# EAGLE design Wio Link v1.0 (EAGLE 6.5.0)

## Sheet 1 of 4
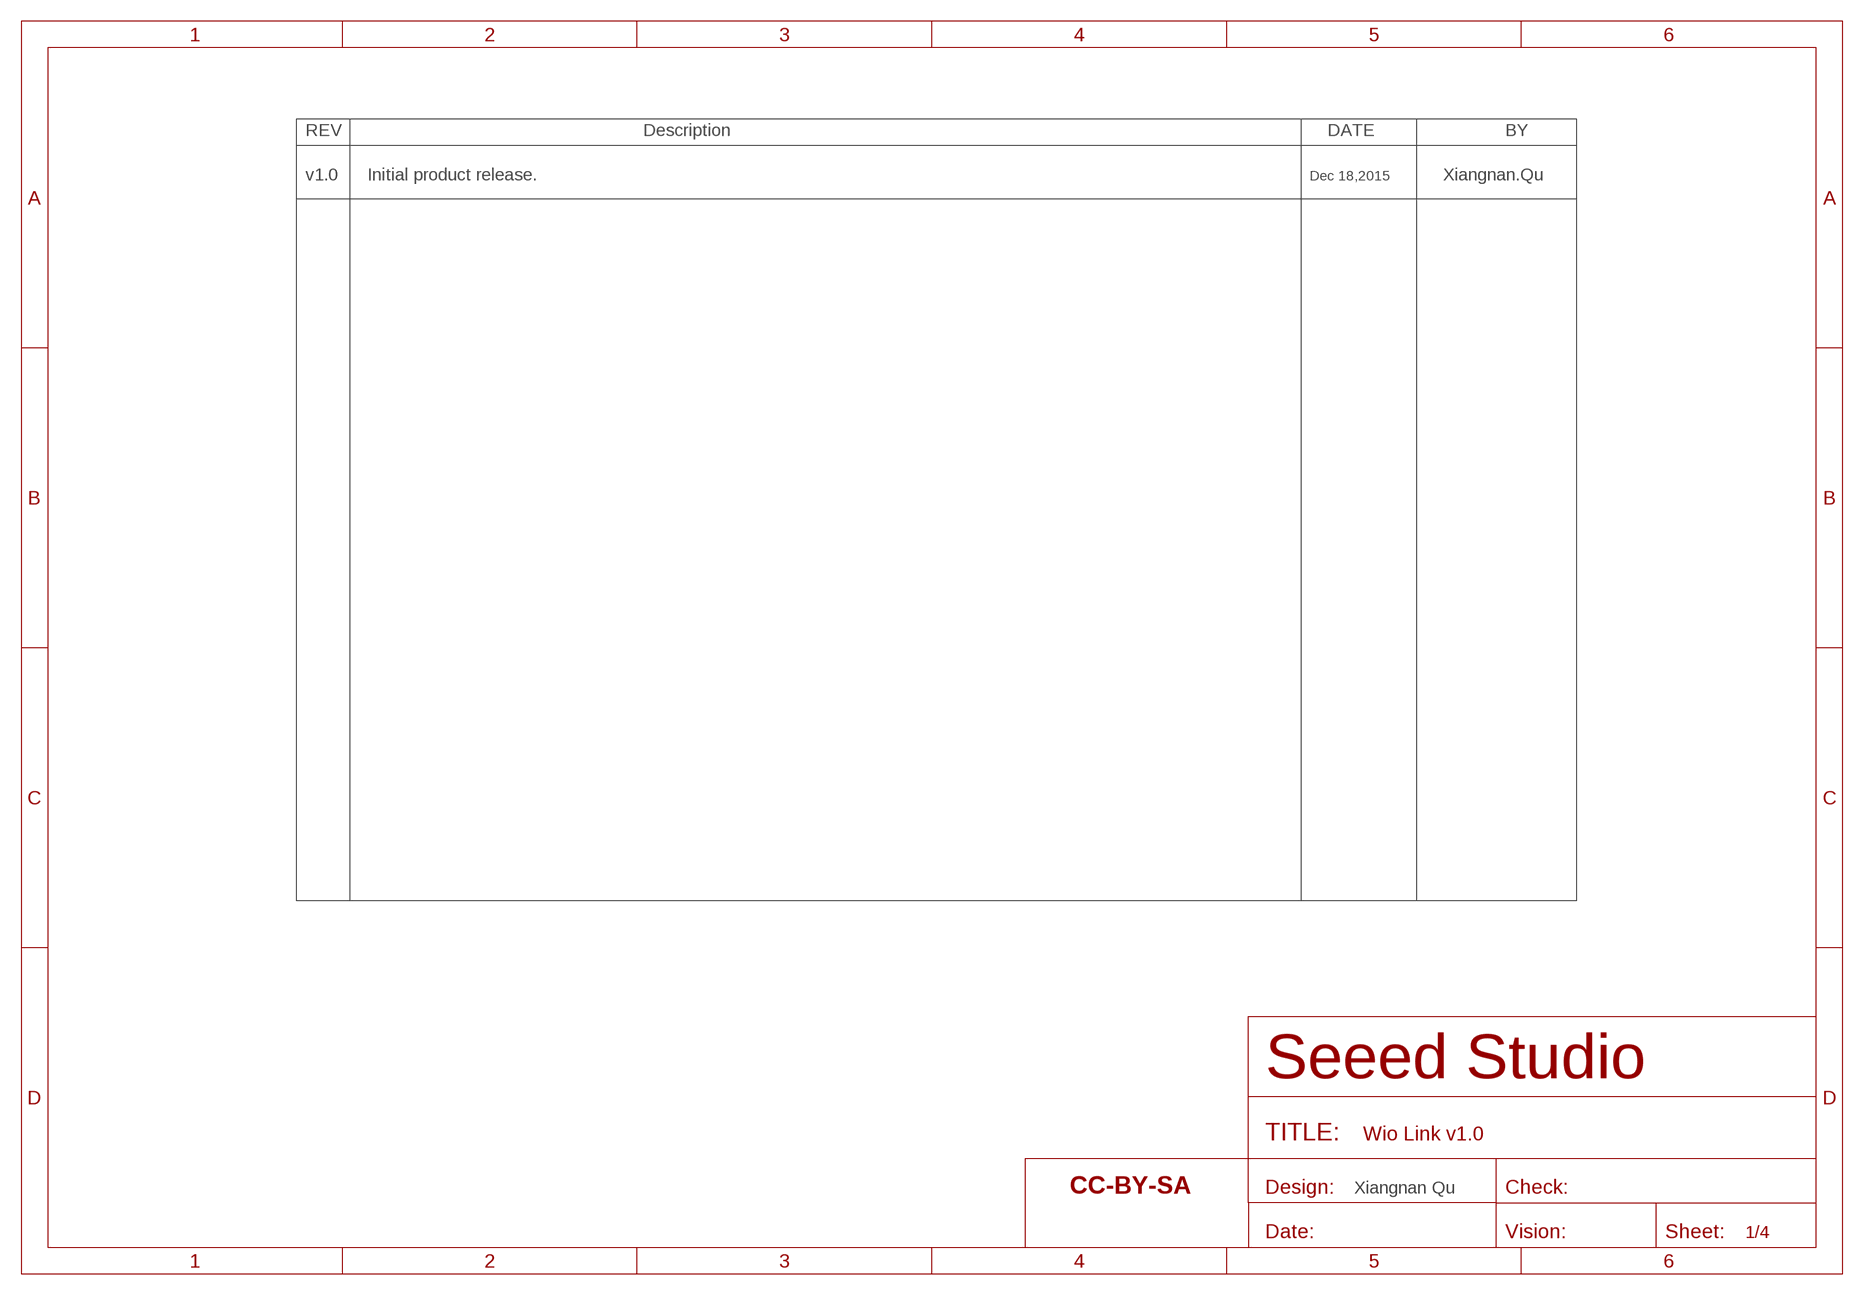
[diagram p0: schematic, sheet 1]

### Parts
FR4  SEEEDSTUDIO-OPEN-SCH-FRAME  [SEEEDSTUDIO-PCB-FRAME]

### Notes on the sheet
- v1.0 | Initial product release. | Dec 18,2015 | Xiangnan.Qu
- Xiangnan Qu

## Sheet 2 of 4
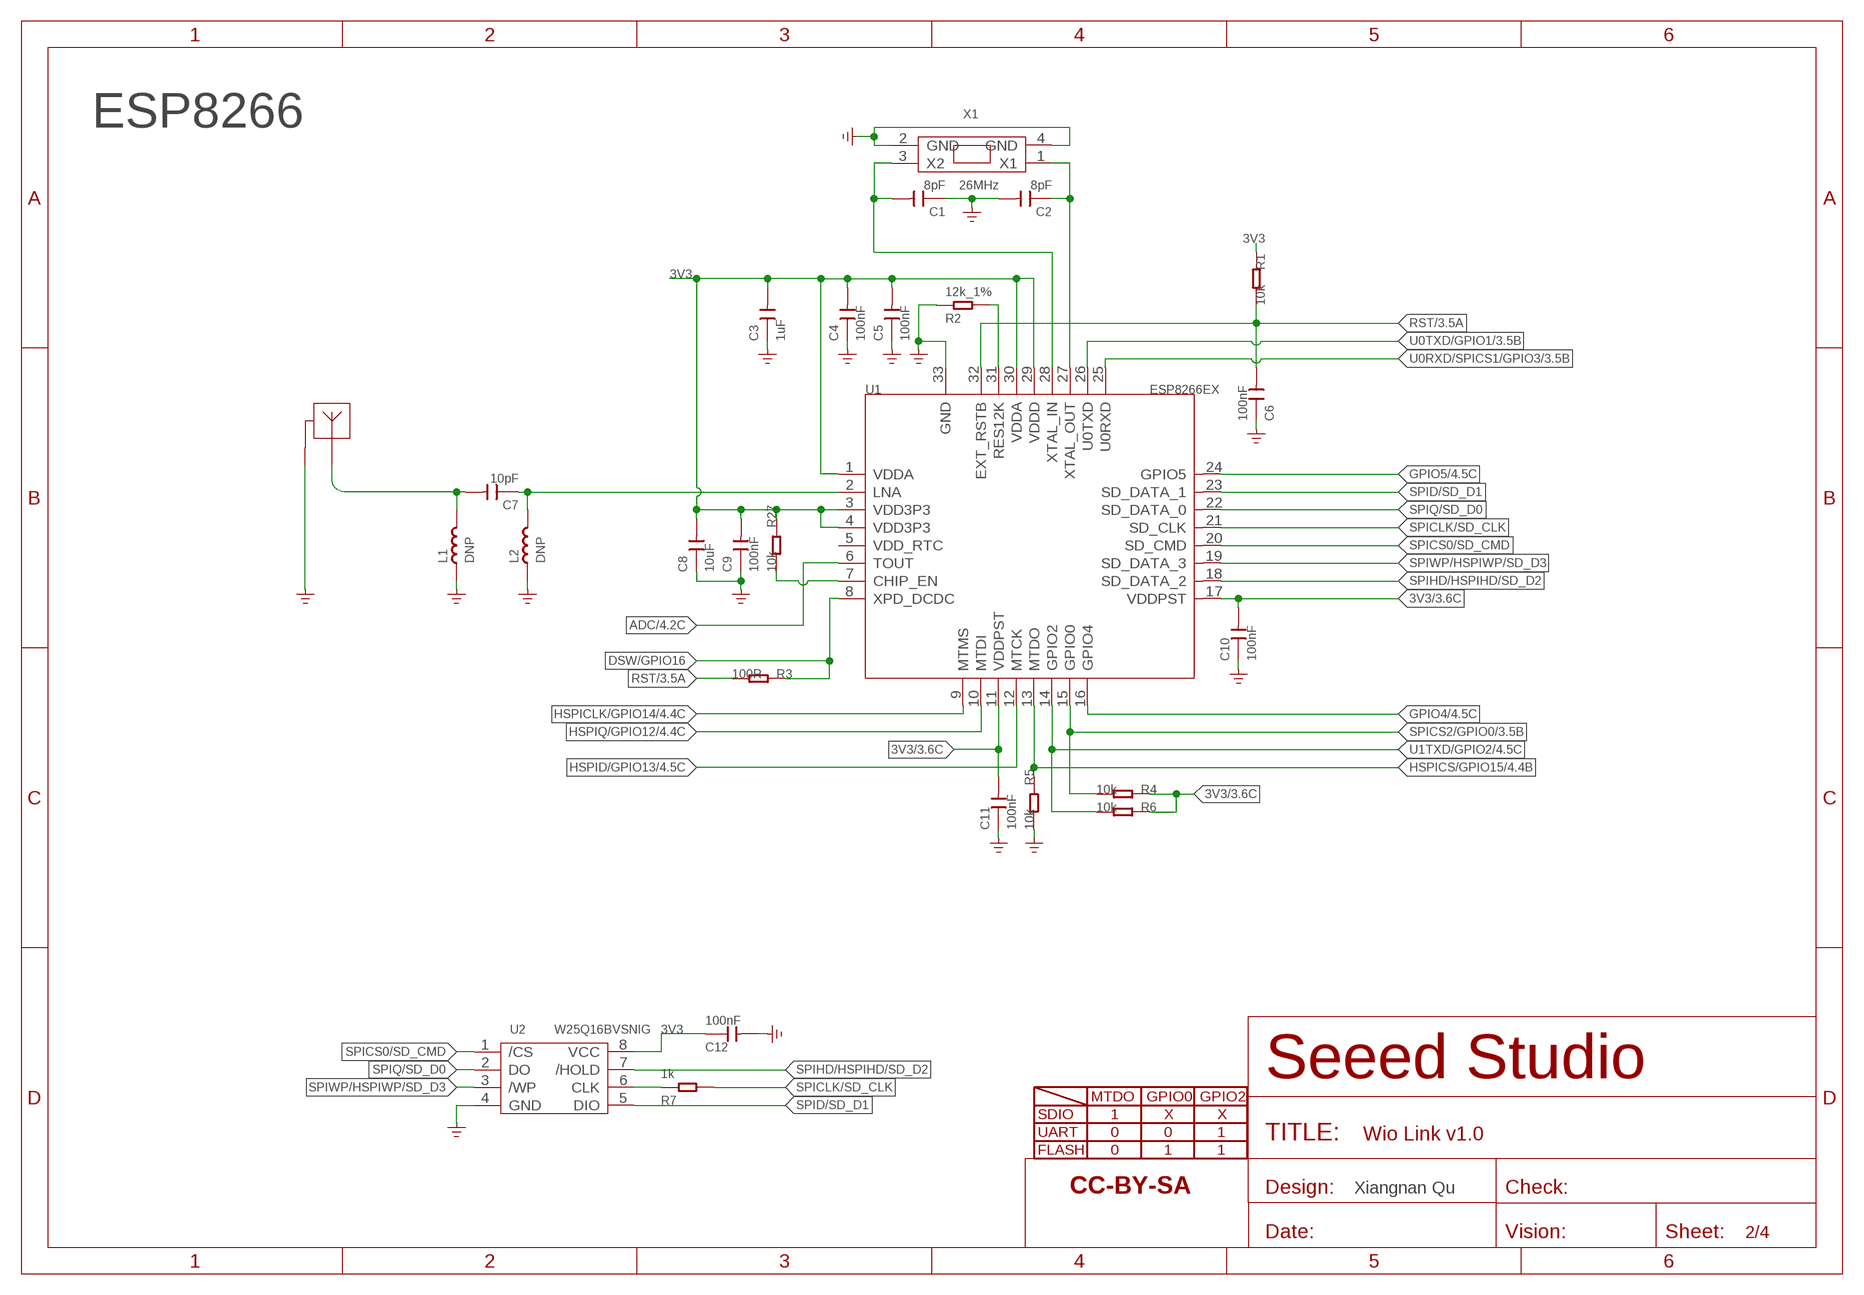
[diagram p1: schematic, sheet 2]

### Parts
ANT1  ANTENNA-2.4G-ANT5  [SWRU120B]
C1  8pF  CAP-0402  [C0402]
C2  8pF  CAP-0402  [C0402]
C3  1uF  CAP-0402  [C0402]
C4  100nF  CAP-0402  [C0402]
C5  100nF  CAP-0402  [C0402]
C6  100nF  CAP-0402  [C0402]
C7  10pF  CAP-0402  [C0402]
C8  10uF  CAP-0603  [C0603]
C9  100nF  CAP-0402  [C0402]
C10  100nF  CAP-0402  [C0402]
C11  100nF  CAP-0402  [C0402]
C12  100nF  CAP-0402  [C0402]
FR1  SEEEDSTUDIO-OPEN-SCH-FRAME  [SEEEDSTUDIO-PCB-FRAME]
L1  DNP  INDUCTOR/FERRITE-BEAD'0402'  [L0402]
L2  DNP  INDUCTOR/FERRITE-BEAD'0402'  [L0402]
R1  10k  RES-0402  [R0402]
R2  12k_1%  RES-0402  [R0402]
R3  100R  RES-0402  [R0402]
R4  10k  RES-0402  [R0402]
R5  10k  RES-0402  [R0402]
R6  10k  RES-0402  [R0402]
R7  1k  RES-0402  [R0402]
R27  10k  RES-0402  [R0402]
U1  ESP8266EX  MOUDLE-WIFI-ESP8266EX-ESP8266  [QFN32G-0.5-5X5MM]
U2  W25Q16BVSNIG  FLASH-W25X80-1.27  [SON8-1.27-5X6MM]
X1  26MHz  CRYSTAL-4P  [X4-SMD-3.2X2.5X0.7MM]

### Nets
3V3: C3.2 C4.2 C5.2 C8.2 C9.2 C10.2 C11.2 C12.1 R1.1 R4.1 R6.1 R27.1 U1.1(VDDA) U1.3(VDD3P3) U1.4(VDD3P3) U1.11(VDDPST) U1.17(VDDPST) U1.29(VDDD) U1.30(VDDA) U2.8(VCC) ; also sheet 3,4
ADC: U1.6(TOUT) ; also sheet 4
DSW/GPIO16: R3.1 U1.8(XPD_DCDC)
GND: ANT1.1 C1.1 C2.2 C3.1 C4.1 C5.1 C6.1 C8.1 C9.1 C10.1 C11.1 C12.2 L1.1 L2.1 R2.2 R5.2 U1.33(GND) U2.4(GND) X1.2(GND) X1.4(GND) ; supply symbol labelled GND_POWER ; also sheet 3,4
GPIO4: U1.16(GPIO4) ; also sheet 4
GPIO5: U1.24(GPIO5) ; also sheet 4
HSPICLK/GPIO14: U1.9(MTMS) ; also sheet 4
HSPICS/GPIO15: R5.1 U1.13(MTDO) ; also sheet 4
HSPID/GPIO13: U1.12(MTCK) ; also sheet 4
HSPIQ/GPIO12: U1.10(MTDI) ; also sheet 4
N$1: R2.1 U1.31(RES12K)
N$2: C1.2 U1.28(XTAL_IN) X1.3(X2)
N$3: C2.1 U1.27(XTAL_OUT) X1.1(X1)
N$4: R27.2 U1.7(CHIP_EN)
N$5: C7.1 L2.2 U1.2(LNA)
N$6: ANT1.2 C7.2 L1.2
N$10: R7.1 U2.6(CLK)
RST: C6.2 R1.2 R3.2 U1.32(EXT_RSTB) ; also sheet 3,4
SPICLK/SD_CLK: R7.2 U1.21(SD_CLK)
SPICS0/SD_CMD: U1.20(SD_CMD) U2.1(/CS)
SPICS2/GPIO0: R4.2 U1.15(GPIO0) ; also sheet 3,4
SPID/SD_D1: U1.23(SD_DATA_1) U2.5(DIO)
SPIHD/HSPIHD/SD_D2: U1.18(SD_DATA_2) U2.7(/HOLD)
SPIQ/SD_D0: U1.22(SD_DATA_0) U2.2(DO)
SPIWP/HSPIWP/SD_D3: U1.19(SD_DATA_3) U2.3(/WP)
U0RXD/SPICS1/GPIO3: U1.25(U0RXD) ; also sheet 3,4
U0TXD/GPIO1: U1.26(U0TXD) ; also sheet 3,4
U1TXD/GPIO2: R6.2 U1.14(GPIO2) ; also sheet 4
Unconnected: U1.5(VDD_RTC)

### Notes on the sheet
- ESP8266
- MTDO | GPIO0 | GPIO2
- SDIO | 1 | X | X
- UART | 0 | 0 | 1
- FLASH | 0 | 1 | 1
- Xiangnan Qu

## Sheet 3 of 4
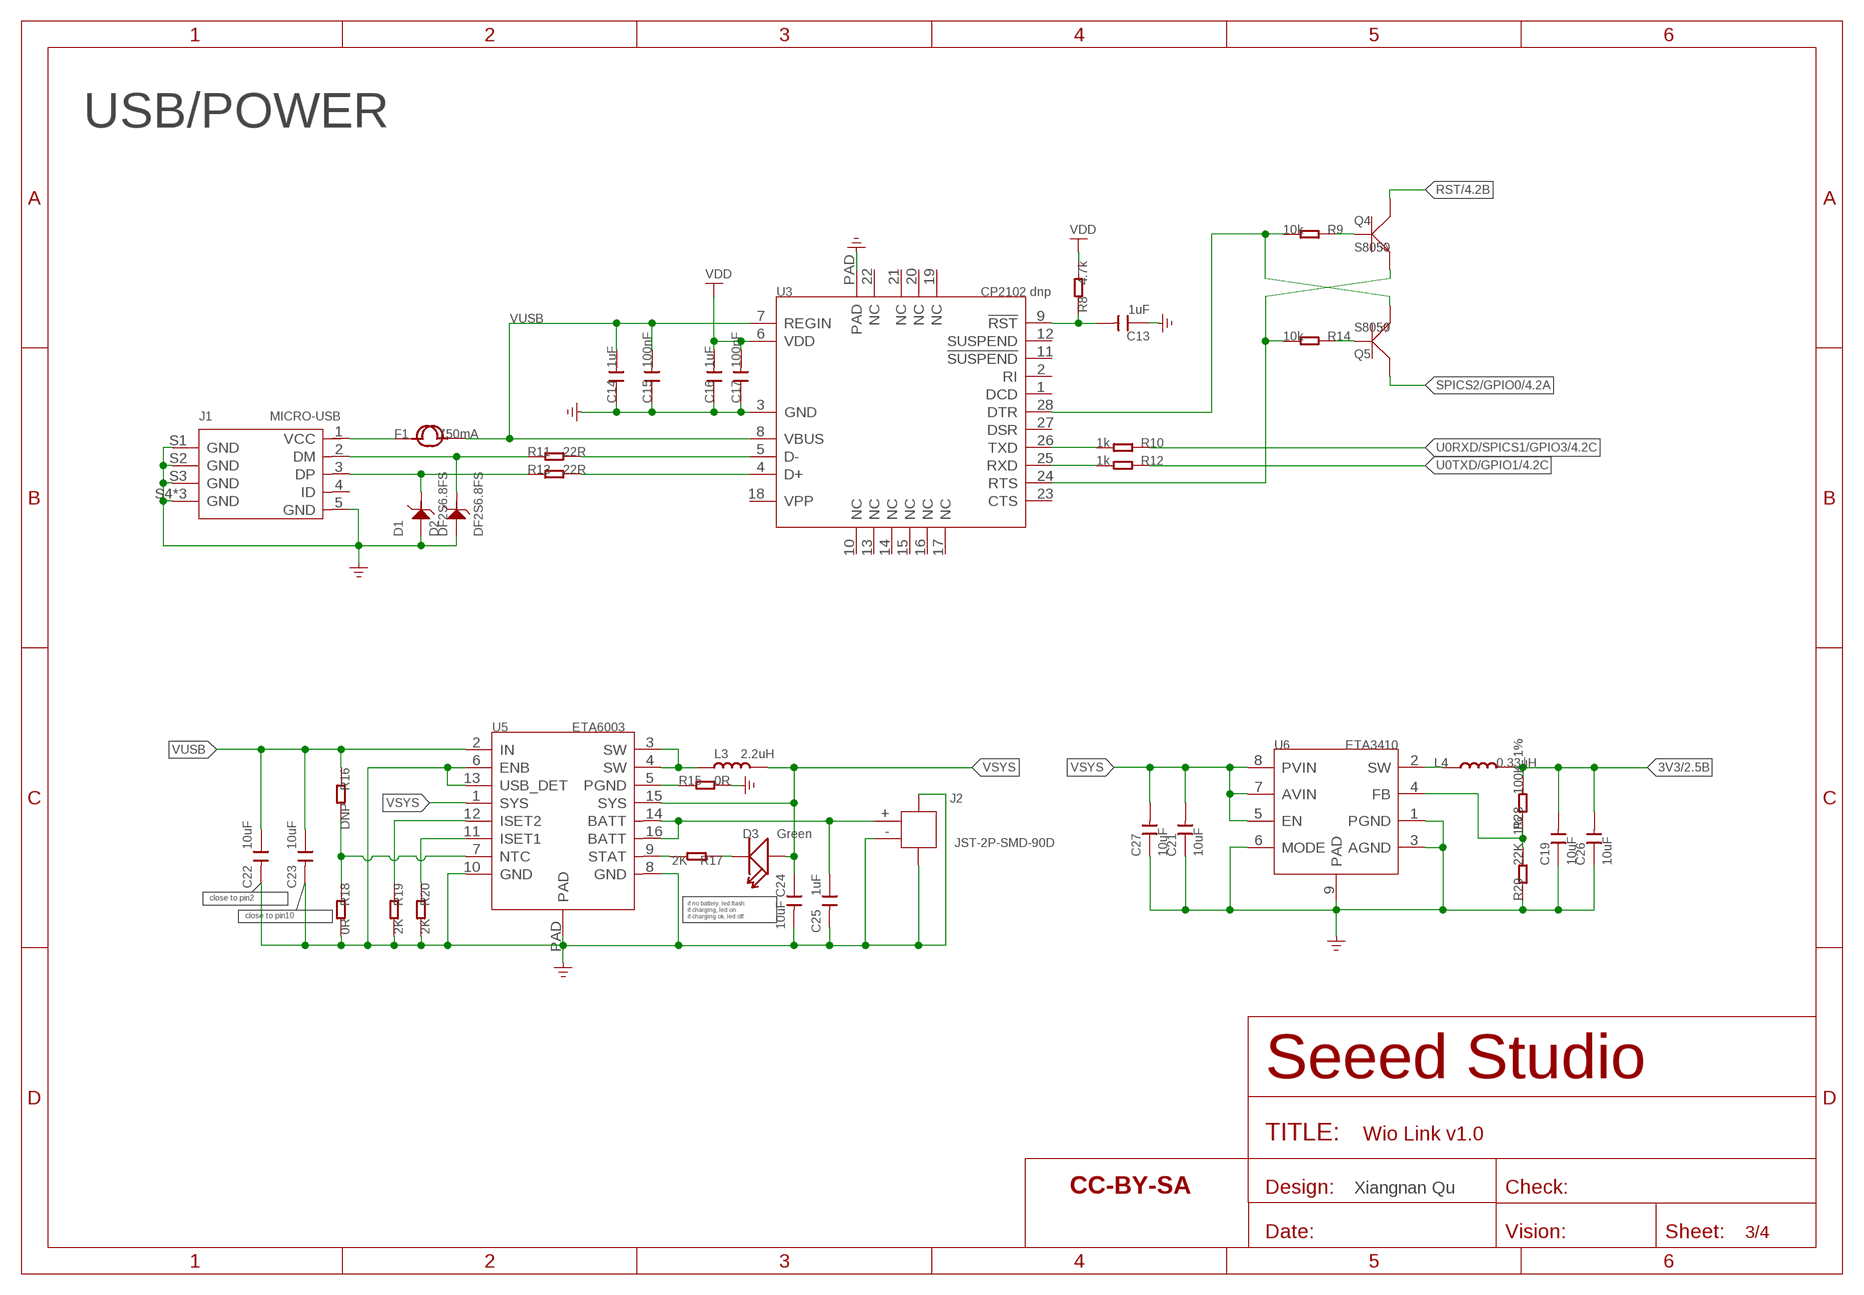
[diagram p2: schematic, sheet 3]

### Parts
C13  1uF  CAP-0402  [C0402]
C14  1uF  CAP-0402  [C0402]
C15  100nF  CAP-0402  [C0402]
C16  1uF  CAP-0402  [C0402]
C17  100nF  CAP-0402  [C0402]
C19  10uF  CAP-0603  [C0603]
C21  10uF  CAP-0603  [C0603]
C22  10uF  CAP-0805  [C0805]
C23  10uF  CAP-0805  [C0805]
C24  10uF  CAP-0805  [C0805]
C25  1uF  CAP-0402  [C0402]
C26  10uF  CAP-0603  [C0603]
C27  10uF  CAP-0603  [C0603]
D1  DF2S6.8FS  D-ESD-2P'DF2S6.8FS'  [SOD-923]
D2  DF2S6.8FS  D-ESD-2P'DF2S6.8FS'  [SOD-923]
D3  Green  LED-0402  [LED-0402]
F1  750mA  FUSE+'1206'  [FS1206]
FR2  SEEEDSTUDIO-OPEN-SCH-FRAME  [SEEEDSTUDIO-PCB-FRAME]
J1  MICRO-USB  MICRO-USB5+4P'5+4P'  [MICRO-USB5+4P-SMD-0.65-B]
J2  JST-2P-SMD-90D  JST-2P-SMD'2.0'  [HW2-SMD-2.0-90D]
L3  2.2uH  INDUCTOR/FERRITE-BEAD'0805'  [L0805]
L4  0.33uH  L-MPM201610SR33_T  [L201610]
Q4  S8050  TRANSISTOR-NPN-SOT23  [SOT-23]
Q5  S8050  TRANSISTOR-NPN-SOT23  [SOT-23]
R8  4.7k  RES-0402  [R0402]
R9  10k  RES-0402  [R0402]
R10  1k  RES-0402  [R0402]
R11  22R  RES-0402  [R0402]
R12  1k  RES-0402  [R0402]
R13  22R  RES-0402  [R0402]
R14  10k  RES-0402  [R0402]
R15  0R  RES-0402  [R0402]
R16  DNP  RES-0402  [R0402]
R17  2K  RES-0402  [R0402]
R18  0R  RES-0402  [R0402]
R19  2K  RES-0402  [R0402]
R20  2K  RES-0402  [R0402]
R28  100K_1%  RES-0402  [R0402]
R29  22K_1%  RES-0402  [R0402]
U3  CP2102 dnp  TRANSFER_CP2102_9  [QFN28]
U5  ETA6003  PMIC-ETA6003  [QFN16G-0.5-3X3MM]
U6  ETA3410  CONVERTER-ETA3410  [DFN8G-0.5-2X2MM]

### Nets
3V3: C19.2 C26.2 L4.2 R28.2 ; also sheet 2,4
GND: C13.1 C14.1 C15.1 C16.1 C17.1 C19.1 C21.1 C22.2 C23.2 C24.2 C25.2 C26.1 C27.1 D1.2 D2.2 J1.5(GND) J1.S1(GND) J1.S2(GND) J1.S3(GND) J1.S4(GND) J1.S5(GND) J1.S6(GND) J2.3 J2.4 J2.- R15.2 R18.2 R19.2 R20.2 R29.1 U3.3(GND) U3.PAD U5.6(ENB) U5.8(GND) U5.10(GND) U5.13(USB_DET) U5.PAD U6.1(PGND) U6.3(AGND) U6.6(MODE) U6.9(PAD) ; supply symbol labelled GND_POWER ; also sheet 2,4
N$8: R10.2 U3.26(TXD)
N$12: F1.1 J1.1(VCC)
N$13: R11.2 U3.5(D-)
N$15: D2.1 J1.2(DM) R11.1
N$16: D1.1 J1.3(DP) R13.1
N$17: R13.2 U3.4(D+)
N$18: Q5.1(B) R14.1
N$19: C13.2 R8.1 U3.9(!RST)
N$20: R12.2 U3.25(RXD)
N$23: Q4.2(E) R14.2 U3.24(RTS)
N$24: Q5.2(E) R9.2 U3.28(DTR)
N$25: Q4.1(B) R9.1
N$26: L3.1 U5.3(SW) U5.4(SW)
N$28: C25.1 J2.+ U5.14(BATT) U5.16(BATT)
N$29: L4.1 U6.2(SW)
N$30: D3.- R17.1
N$31: R17.2 U5.9(STAT)
N$32: R28.1 R29.2 U6.4(FB)
N$33: R16.2 R18.1 U5.7(NTC)
N$34: R20.1 U5.11(ISET1)
N$36: R19.1 U5.12(ISET2)
N$37: R15.1 U5.5(PGND)
RST: Q4.3(C) ; also sheet 2,4
SPICS2/GPIO0: Q5.3(C) ; also sheet 2,4
U0RXD/SPICS1/GPIO3: R10.1 ; also sheet 2,4
U0TXD/GPIO1: R12.1 ; also sheet 2,4
VDD: C16.2 C17.2 R8.2 U3.6(VDD) ; supply symbol labelled POWER_BAR
VSYS: C21.2 C24.1 C27.2 D3.+ L3.2 U5.1(SYS) U5.15(SYS) U6.5(EN) U6.7(AVIN) U6.8(PVIN)
VUSB: C14.2 C15.2 C22.1 C23.1 F1.2 R16.1 U3.7(REGIN) U3.8(VBUS) U5.2(IN)
Unconnected: J1.4(ID) U3.1(DCD) U3.2(RI) U3.10(NC) U3.11(!SUSPEND) U3.12(SUSPEND) U3.13(NC) U3.14(NC) U3.15(NC) U3.16(NC) U3.17(NC) U3.18(VPP) U3.19(NC) U3.20(NC) U3.21(NC) U3.22(NC) U3.23(CTS) U3.27(DSR)

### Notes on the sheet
- USB/POWER
- close to pin2
- close to pin10
- if no battery, led flash.
  if charging, led on.
  if charging ok, led off.
- Xiangnan Qu

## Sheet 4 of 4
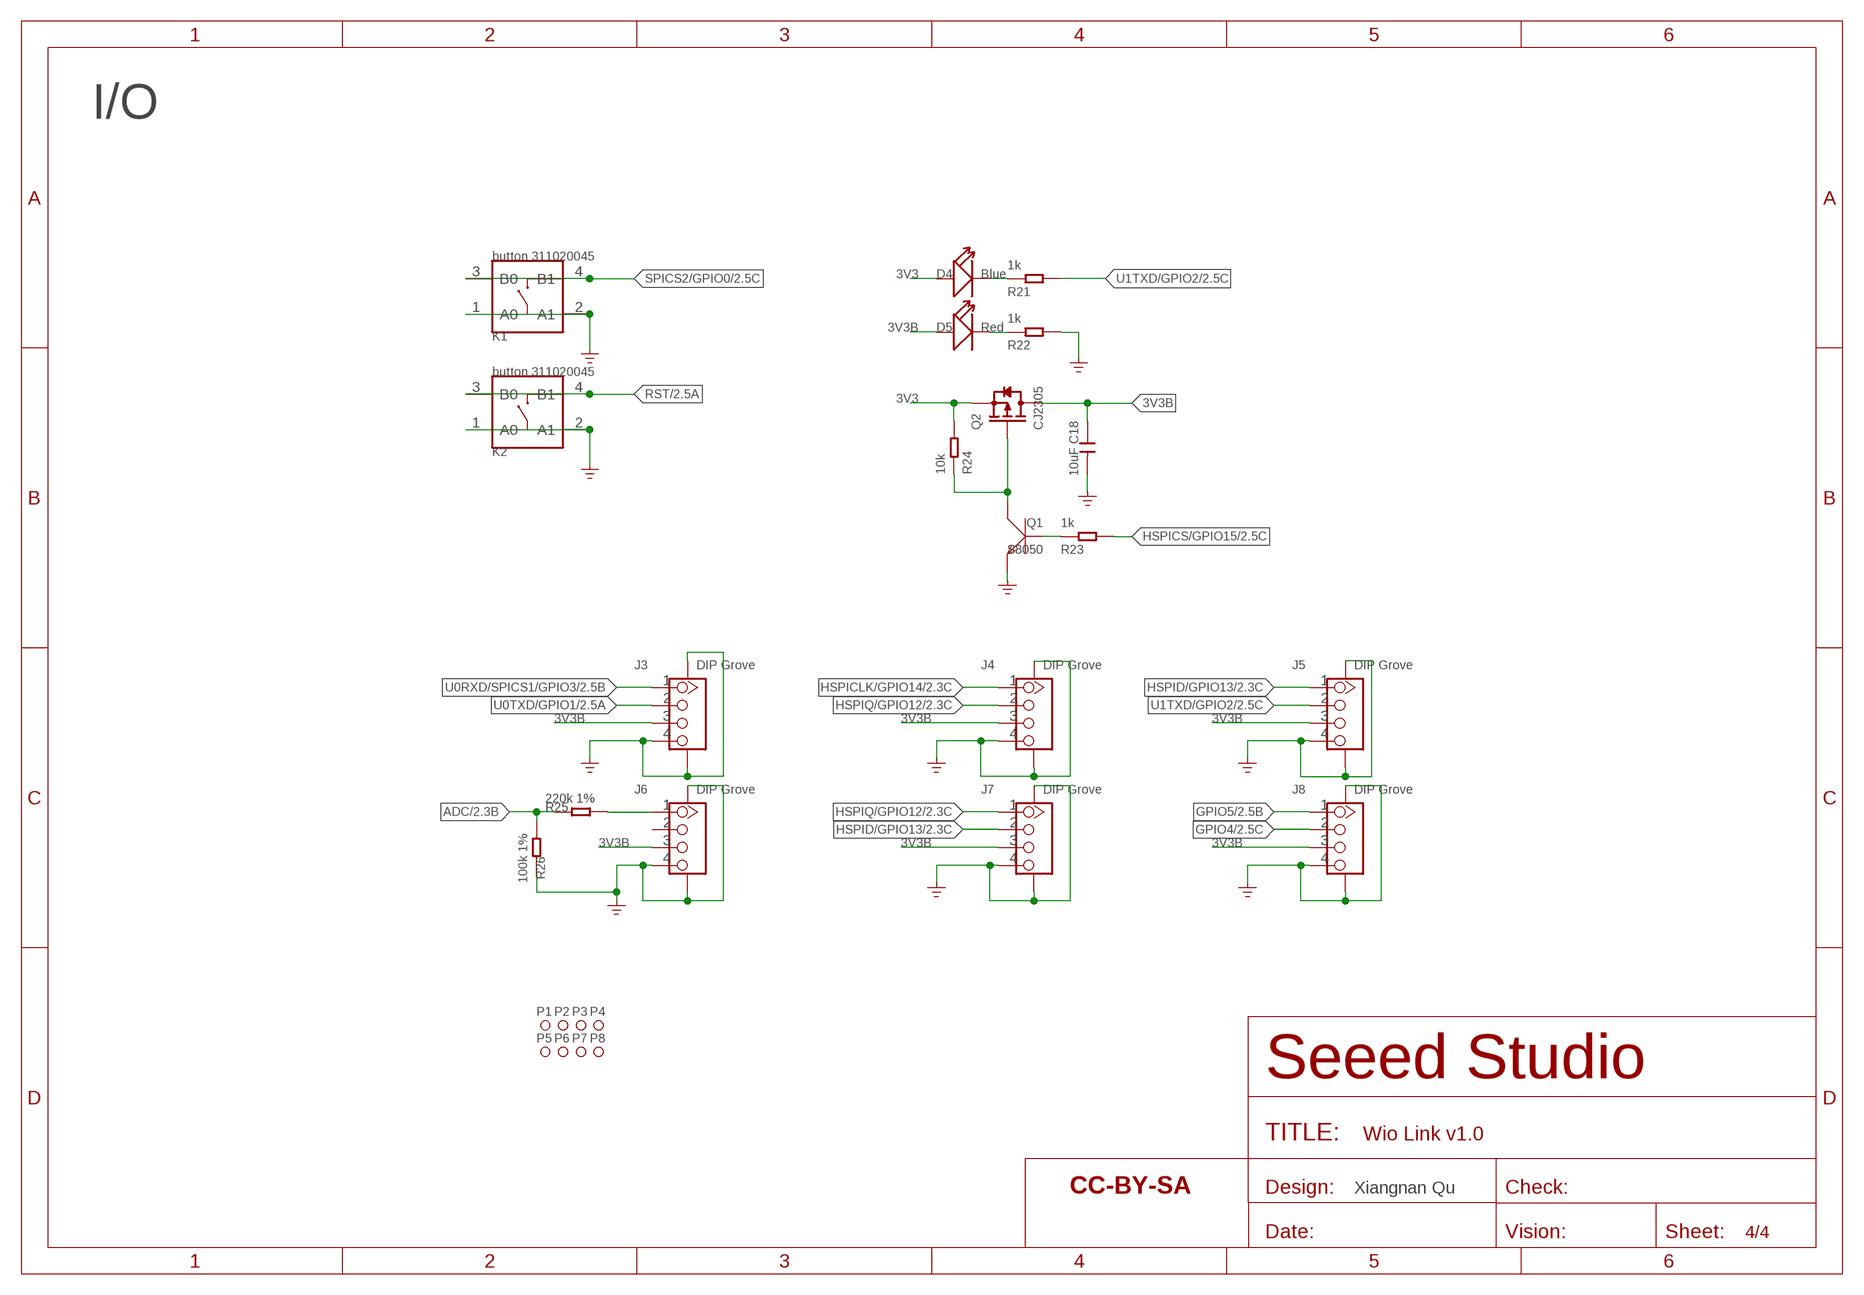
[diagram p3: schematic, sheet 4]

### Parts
C18  10uF  CAP-0805  [C0805]
D4  Blue  LED'0603'  [LED-0603]
D5  Red  LED'0603'  [LED-0603]
FR3  SEEEDSTUDIO-OPEN-SCH-FRAME  [SEEEDSTUDIO-PCB-FRAME]
J3  DIP Grove  GROVE-CONNECTOR-SMD'90D'  [HW4-SMD-2.0-90D]
J4  DIP Grove  GROVE-CONNECTOR-SMD'90D'  [HW4-SMD-2.0-90D]
J5  DIP Grove  GROVE-CONNECTOR-SMD'90D'  [HW4-SMD-2.0-90D]
J6  DIP Grove  GROVE-CONNECTOR-SMD'90D'  [HW4-SMD-2.0-90D]
J7  DIP Grove  GROVE-CONNECTOR-SMD'90D'  [HW4-SMD-2.0-90D]
J8  DIP Grove  GROVE-CONNECTOR-SMD'90D'  [HW4-SMD-2.0-90D]
K1  button 311020045  BUTTON-4P-4.5X3.2  [SW4P-SMD-4.5X3.2X2.5MM]
K2  button 311020045  BUTTON-4P-4.5X3.2  [SW4P-SMD-4.5X3.2X2.5MM]
P1  MARK-1.0'ANNULAR'  [ROUND-MARK-1.0]
P2  MARK-1.0'ANNULAR'  [ROUND-MARK-1.0]
P3  MARK-1.0'ANNULAR'  [ROUND-MARK-1.0]
P4  MARK-1.0'ANNULAR'  [ROUND-MARK-1.0]
P5  MARK-1.0'ANNULAR'  [ROUND-MARK-1.0]
P6  MARK-1.0'ANNULAR'  [ROUND-MARK-1.0]
P7  MARK-1.0'ANNULAR'  [ROUND-MARK-1.0]
P8  MARK-1.0'ANNULAR'  [ROUND-MARK-1.0]
Q1  S8050  TRANSISTOR-NPN-SOT23  [SOT-23]
Q2  CJ2305  MOSFET-P'SI2323CDS/SI2305DS<BR>'  [SOT-23]
R21  1k  RES-0402  [R0402]
R22  1k  RES-0402  [R0402]
R23  1k  RES-0402  [R0402]
R24  10k  RES-0402  [R0402]
R25  220k 1%  RES-0402  [R0402]
R26  100k 1%  RES-0402  [R0402]

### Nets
3V3: D4.+ Q2.2(S) R24.2 ; also sheet 2,3
3V3B: C18.1 D5.+ J3.3 J4.3 J5.3 J6.3 J7.3 J8.3 Q2.3(D)
ADC: R25.1 R26.2 ; also sheet 2
GND: C18.2 J3.4 J3.SS1 J3.SS2 J4.4 J4.SS1 J4.SS2 J5.4 J5.SS1 J5.SS2 J6.4 J6.SS1 J6.SS2 J7.4 J7.SS1 J7.SS2 J8.4 J8.SS1 J8.SS2 K1.1(A0) K1.2(A1) K2.1(A0) K2.2(A1) Q1.2(E) R22.2 R26.1 ; supply symbol labelled GND_POWER ; also sheet 2,3
GPIO4: J8.2 ; also sheet 2
GPIO5: J8.1 ; also sheet 2
HSPICLK/GPIO14: J4.1 ; also sheet 2
HSPICS/GPIO15: R23.2 ; also sheet 2
HSPID/GPIO13: J5.1 J7.2 ; also sheet 2
HSPIQ/GPIO12: J4.2 J7.1 ; also sheet 2
N$7: Q1.3(C) Q2.1(G) R24.1
N$9: J6.1 R25.2
N$11: Q1.1(B) R23.1
N$14: D4.- R21.1
N$22: D5.- R22.1
RST: K2.3(B0) K2.4(B1) ; also sheet 2,3
SPICS2/GPIO0: K1.3(B0) K1.4(B1) ; also sheet 2,3
U0RXD/SPICS1/GPIO3: J3.1 ; also sheet 2,3
U0TXD/GPIO1: J3.2 ; also sheet 2,3
U1TXD/GPIO2: J5.2 R21.2 ; also sheet 2
Unconnected: J6.2

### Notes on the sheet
- I/O
- Xiangnan Qu

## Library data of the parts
ANT1 = template:ANTENNA-2.4G-ANT
C1-C19 C21-C27 = Discrete-new:CAP: Ceramic Capacitors
D1 D2 = Discrete-new:D-ESD-2P: SOD-923:304060009;SOD-123:304060001
D3-D5 = Discrete-new:LED
F1 = Discrete-new:FUSE+
FR1-FR4 = moudle-new:SEEEDSTUDIO-OPEN-SCH-FRAME
J1 = Connector-new:MICRO-USB5+4P: 5+4P-SMD-0.65-B:320010000;5+2P-SMD-0.65-AB:340032001
J2 = Connector-new:JST-2P-SMD: 2P-SMD-1.0-90D:320110054;2P-SMD-2.0-90D:320110026
J3-J8 = Connector-new:GROVE-CONNECTOR-SMD: 4P-SMD-2.0:320110030;4P-SMD-2.0-90D:320110032
K1 K2 = Discrete-new:BUTTON-4P: SW4-6.0X6.0X5.0MM:311020024;SW4-8.0X8.0X9.0MM:311020028;SW4-SMD-6.0X6.0X5.0MM:311020004;SW4-SMD-3.35X3.35X1.5MM:311020030;SW4-SMD-5.2X5.2X2.5MM:311020046
L1-L3 = Discrete-new:INDUCTOR/FERRITE-BEAD
L4 = Discrete-new:L
P1-P8 = Discrete-new:MARK-1.0; PARTNO: DNP
Q1 Q4 Q5 = Discrete-new:TRANSISTOR-NPN: NPN audion
Q2 = Discrete-new:MOSFET-P
R1-R29 = Discrete-new:RES
U1 = template:MOUDLE-WIFI-ESP8266EX: ESP8266 is complete and ⾃ into system wi-fi ⺴ collaterals solve ⽅ case, should be able to pick up software ⽤, or through the other ⼀ should ⽤ processing
U2 = template:FLASH-W25X80: 1M-BIT,2M-BIT,4M-BIT AND 8M-BIT SERIAL FLASH MEMORY WITH 4KB SECTORS AND DUAL OUTPUT SPI
U3 = template:TRANSFER_CP2102_9
U5 = template:PMIC-ETA6003: 2.5A,3MHZ Switching Charger with Dynamic Power Path Management
U6 = template:CONVERTER-ETA3410: 3MHZ 2A High Step-Down Converter in DFN2x2-8L Package
X1 = Discrete-new:CRYSTAL-4P

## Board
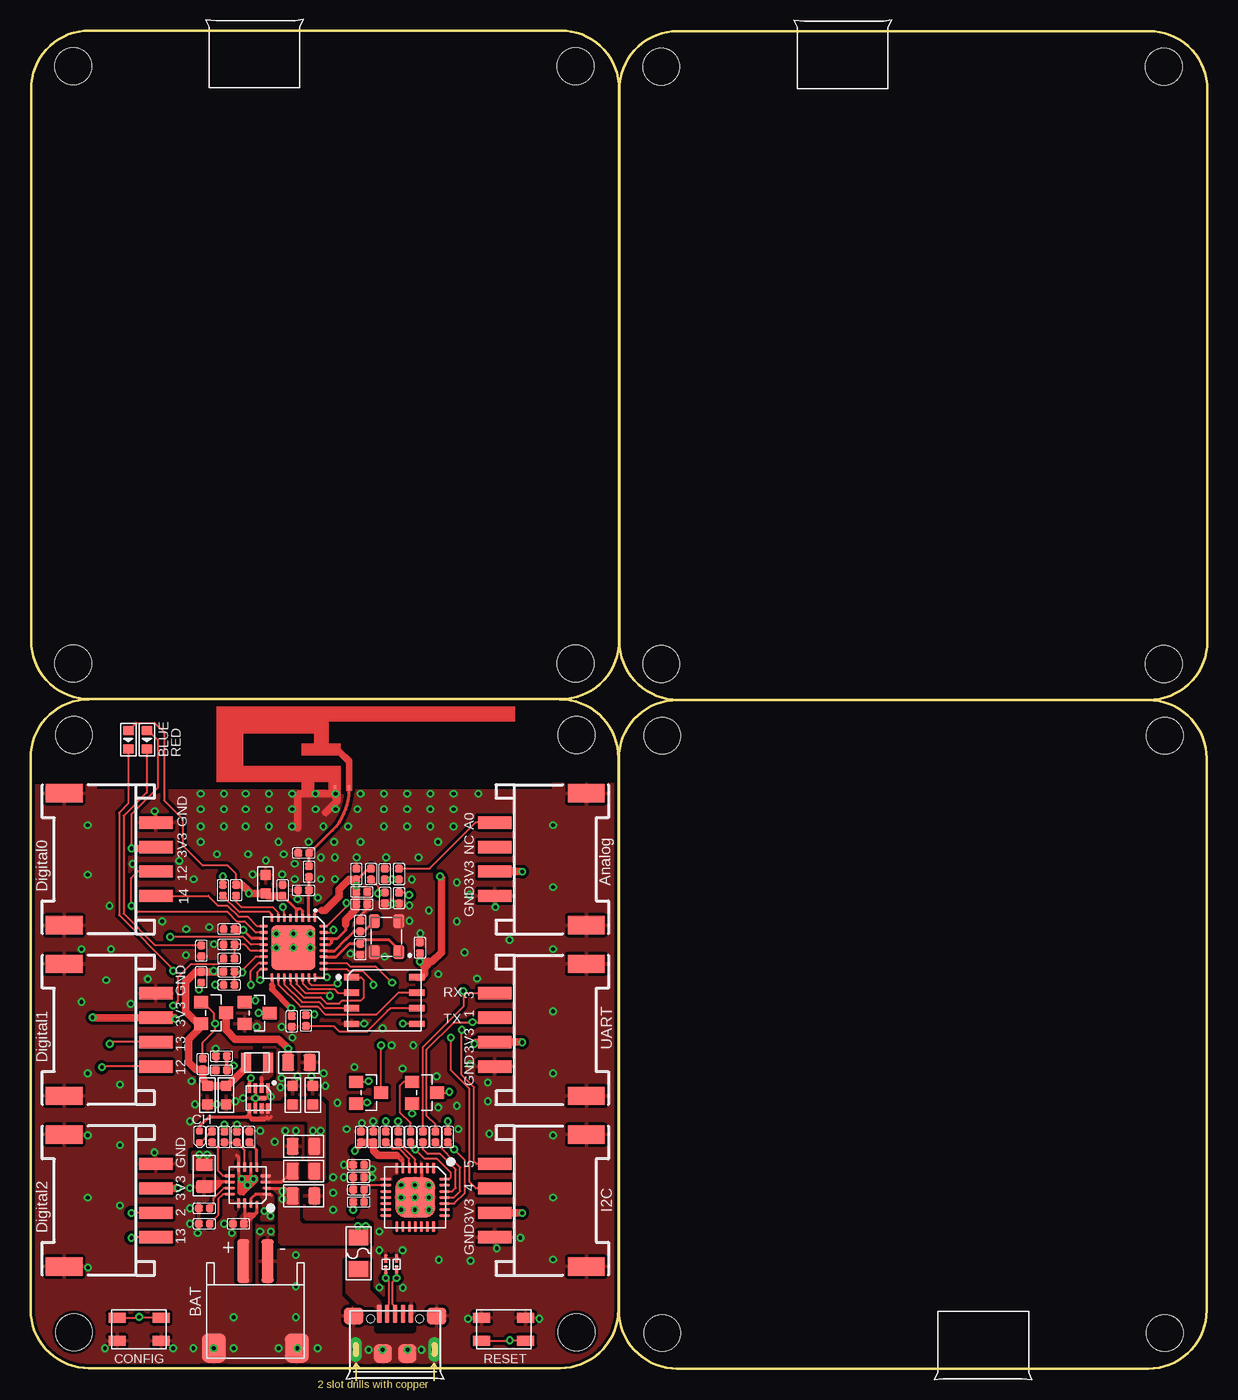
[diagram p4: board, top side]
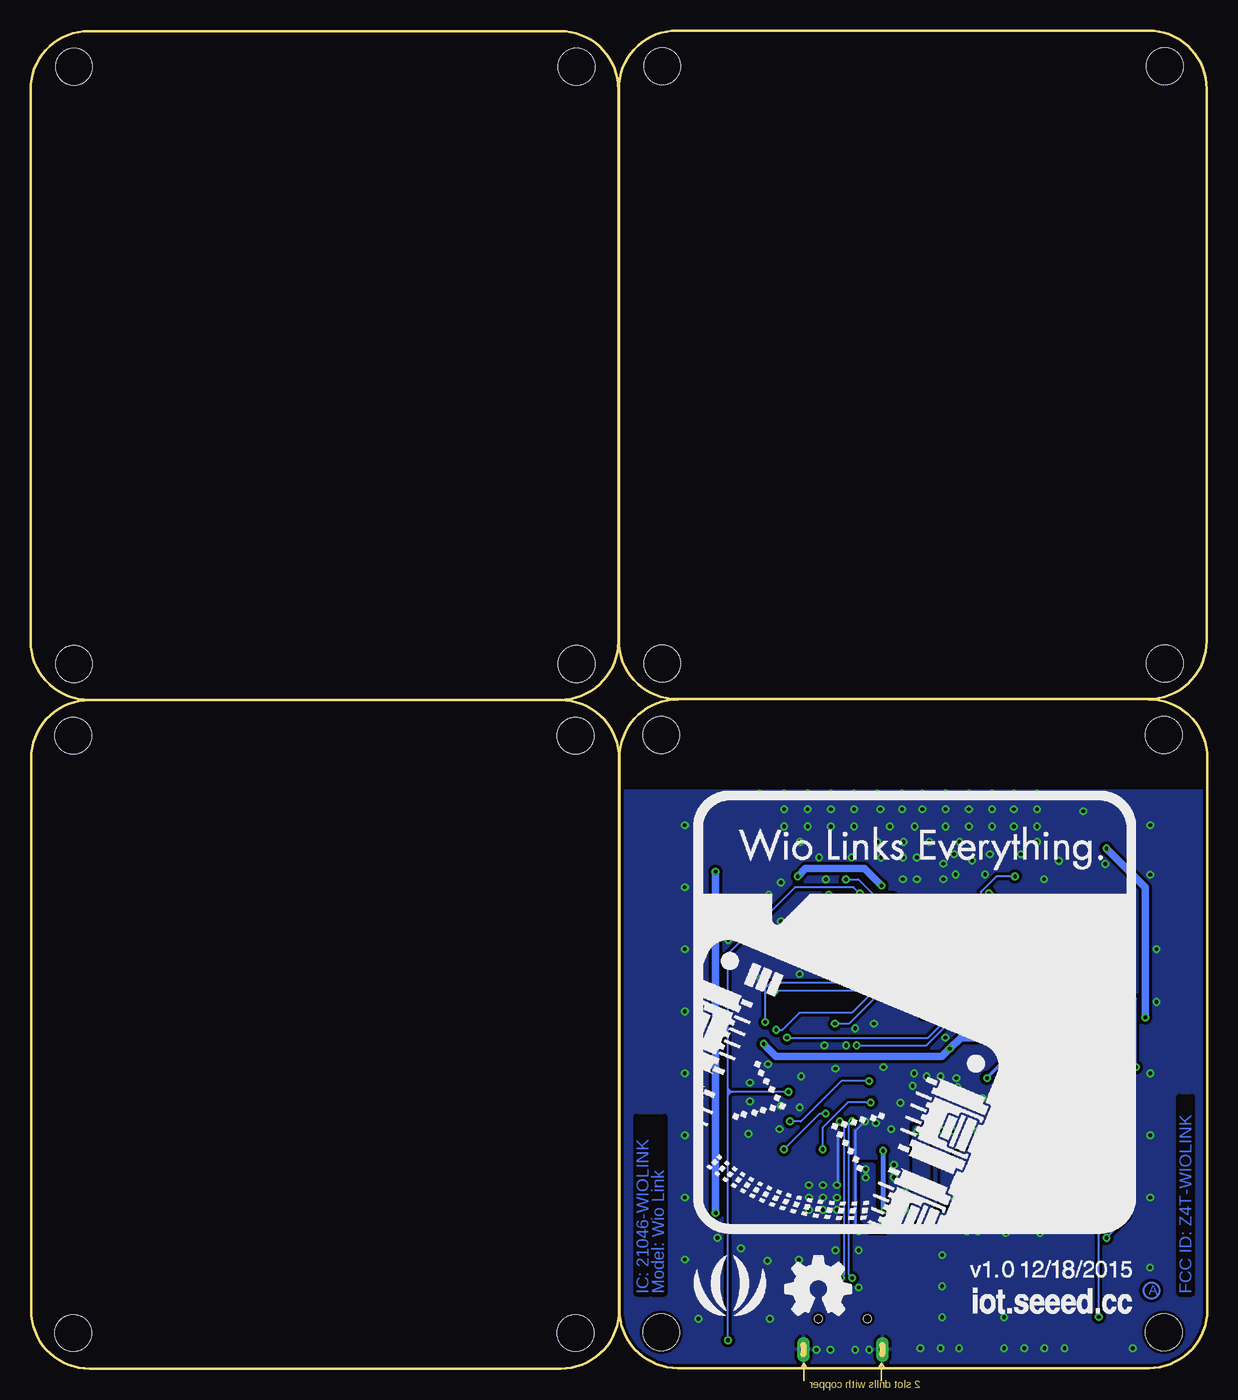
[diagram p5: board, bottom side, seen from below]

Size 96.34 x 109.55 mm. Coordinates in mm from the lower left corner, seen from the top.
Outline: 43.35,54.79 arc-90 48.13,50.01 48.13,4.83 arc-90 43.35,0.05 4.78,0.05 arc-90 0,4.83 0,50.01 arc-90 4.78,54.79
Outline: 48.16,49.96 48.16,4.78 arc90 52.94,0 91.51,0 arc90 96.29,4.78 96.29,49.96 arc90 91.51,54.74 52.94,54.74 arc90 48.16,49.96
Outline: 96.34,59.54 96.34,104.72 arc90 91.56,109.5 52.99,109.5 arc90 48.21,104.72 48.21,59.54 arc90 52.99,54.76 91.56,54.76 arc90 96.34,59.54
Outline: 48.18,59.59 48.18,104.77 arc90 43.4,109.55 4.83,109.55 arc90 0.05,104.77 0.05,59.59 arc90 4.83,54.81 43.4,54.81 arc90 48.18,59.59
Copper layers (1*16): Top 0.035mm / dielectric 1.5mm / Bottom 0.035mm
Design rules "SeeedStudio_2layer_DRU_no_angle_20140221 *": minimum track width 1mil, minimum drill 12mil, track to track 6mil, track to pad 6mil, pad to pad 6mil, via to via 6mil, smd to smd 0mil, copper to edge 10mil, drill to drill 10mil, minimum pad ring 10mil, minimum via ring 6mil, stop-mask expansion 2mil, vias tented up to drill 25mil, thermal gap 10mil
Holes 3 mm at 3.56,2.97 44.7,2.97 3.56,51.87 44.7,51.87 51.71,2.92 92.86,2.92 51.71,51.82 92.86,51.82 92.79,106.58 51.64,106.58 92.79,57.68 51.64,57.68 44.63,106.63 3.48,106.63 44.63,57.73 3.48,57.73
Holes 2 mm at -4.45,2.34 -4.45,107.75 100.97,107.75 100.97,2.34
tRestrict: area 18.4,24.6 to 18.8,26.1
bRestrict: area 1.3,6.1 to 2.3,22.3; area 44.5,6.1 to 46.7,20.6

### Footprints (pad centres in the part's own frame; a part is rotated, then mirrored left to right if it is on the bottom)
SWRU120B = smd 0.203 x 0.406: 1 -0.5,0.26; 2 0.68,0.26
C0402 = smd 0.635 x 0.635: 1 0,0.445; 2 0,-0.445
C0603 = smd 0.889 x 0.889: 1 0,0.762; 2 0,-0.762
C0805 = smd 1.397 x 1.016: 1 0,0.889; 2 0,-0.889
SOD-923 = smd 0.7 x 0.3: 1 -0.45,0; 2 0.45,0
LED-0402 = smd 0.58 x 0.58: + -0.468,0; - 0.468,0
LED-0603 = smd 0.762 x 0.889: + -0.762,0; - 0.762,0
FS1206 = smd 1.27 x 1.524: 1 -1.27,0; 2 1.27,0
MICRO-USB5+4P-SMD-0.65-B = smd 0.381 x 1.524: 1 -1.3,-0.25; 2 -0.65,-0.25; 3 0,-0.25; 4 0.65,-0.25; 5 1.3,-0.25 | smd 1.6 x 1.397: S1 -3.4,-0.427; S6 3.4,-0.427 | drill 0.508 pad 1.016 long: S2 -3.226,-3.175; S5 3.226,-3.175 | smd 1.5 x 1.5: S3 -1,-3.5; S4 1,-3.5 | hole 0.635: -2,-0.65; 2,-0.65
HW2-SMD-2.0-90D = smd 2 x 2.4: 3 3.4,-2.181; 4 -3.4,-2.181 | smd 1 x 3.6: + -1,4.953; - 1,4.953
HW4-SMD-2.0-90D = smd 1.01 x 2.74: 1 -3,-0.1; 2 -1,-0.1; 3 1,-0.1; 4 3,-0.1 | smd 1.5 x 3: SS1 -5.4,7.4; SS2 5.4,7.4
SW4P-SMD-4.5X3.2X2.5MM = smd 1.4 x 0.8: 1 -1.8,-0.94; 2 1.8,-0.94; 3 1.8,0.94; 4 -1.8,0.94
L0402 = smd 0.635 x 0.635: 1 -0.445,0; 2 0.445,0
L0805 = smd 1.016 x 1.397: 1 -0.889,0; 2 0.889,0
L201610 = smd 0.8 x 1.6: 1 -0.9,0; 2 0.9,0
ROUND-MARK-1.0 = smd 1.016 x 1.016: P$1 0,0
SOT-23 = smd 1.016 x 1.143: 1 -0.889,-1.016; 2 0.889,-1.016; 3 0,1.016
R0402 = smd 0.635 x 0.635: 1 0,0.445; 2 0,-0.445
QFN32G-0.5-5X5MM = smd 0.7 x 0.25: 1 -2.45,1.75; 2 -2.45,1.25; 3 -2.45,0.75; 4 -2.45,0.25; 5 -2.45,-0.25; 6 -2.45,-0.75; 7 -2.45,-1.25; 8 -2.45,-1.75; 17 2.45,-1.75; 18 2.45,-1.25; 19 2.45,-0.75; 20 2.45,-0.25; 21 2.45,0.25; 22 2.45,0.75; 23 2.45,1.25; 24 2.45,1.75 | smd 0.25 x 0.7: 9 -1.75,-2.45; 10 -1.25,-2.45; 11 -0.75,-2.45; 12 -0.25,-2.45; 13 0.25,-2.45; 14 0.75,-2.45; 15 1.25,-2.45; 16 1.75,-2.45; 25 1.75,2.45; 26 1.25,2.45; 27 0.75,2.45; 28 0.25,2.45; 29 -0.25,2.45; 30 -0.75,2.45; 31 -1.25,2.45; 32 -1.75,2.45 | smd 3.6 x 3.6: 33 0,0
SON8-1.27-5X6MM = smd 0.5 x 1.25: 1 -1.905,-2.675; 2 -0.635,-2.675; 3 0.635,-2.675; 4 1.905,-2.675; 5 1.905,2.675; 6 0.635,2.675; 7 -0.635,2.675; 8 -1.905,2.675
QFN28 = smd 0.9 x 0.25: 1 -2.4,1.5; 2 -2.4,1; 3 -2.4,0.5; 4 -2.4,0; 5 -2.4,-0.5; 6 -2.4,-1; 7 -2.4,-1.5; 15 2.4,-1.5; 16 2.4,-1; 17 2.4,-0.5; 18 2.4,0; 19 2.4,0.5; 20 2.4,1; 21 2.4,1.5 | smd 0.25 x 0.9: 8 -1.5,-2.4; 9 -1,-2.4; 10 -0.5,-2.4; 11 0,-2.4; 12 0.5,-2.4; 13 1,-2.4; 14 1.5,-2.4; 22 1.5,2.4; 23 1,2.4; 24 0.5,2.4; 25 0,2.4; 26 -0.5,2.4; 27 -1,2.4; 28 -1.5,2.4 | smd 3.25 x 3.25: PAD 0,0
QFN16G-0.5-3X3MM = smd 0.65 x 0.28: 1 -1.575,0.75; 2 -1.575,0.25 | smd 0.85 x 0.28: 3 -1.475,-0.25; 4 -1.475,-0.75; 9 1.475,-0.75; 10 1.475,-0.25; 11 1.475,0.25; 12 1.475,0.75 | smd 0.28 x 0.85: 5 -0.75,-1.475; 6 -0.25,-1.475; 7 0.25,-1.475; 8 0.75,-1.475; 13 0.75,1.475; 14 0.25,1.475 | smd 0.28 x 0.65: 15 -0.25,1.575; 16 -0.75,1.575 | smd 0.508 x 0.508: PAD 0,0
DFN8G-0.5-2X2MM = smd 0.8 x 0.3: 1 -0.827,0.75; 2 -0.827,0.25; 3 -0.827,-0.25; 4 -0.827,-0.75; 5 0.827,-0.75; 6 0.827,-0.25; 7 0.827,0.25; 8 0.827,0.75 | smd 0.45 x 1.3: 9 0,0
X4-SMD-3.2X2.5X0.7MM = smd 1.143 x 0.889: 1 -1.27,-1.016; 2 1.27,-1.016; 3 1.27,1.016; 4 -1.27,1.016

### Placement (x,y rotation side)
ANT1  25.4,47.29 0 top
C1  26.99,36.25 0 top
C2  26.99,34.34 0 top
C3  26.67,40.5 0 top
C4  27.11,38.02 270 top
C5  27.11,39.04 270 top
C6  29.02,38.54 180 top
C7  22.8,40.69 180 top
C8  19.24,39.67 0 top
C9  20.64,39.17 0 top
C10  21.39,28.44 180 top
C11  16.26,35.99 90 top
C12  31.88,34.47 180 top
C13  26.86,14.66 90 top
C14  26.86,15.67 90 top
C15  26.86,16.69 90 top
C16  27.05,18.97 0 top
C17  28.07,18.97 0 top
C18  21.97,25.07 90 top
C19  16,22.4 180 top
C21  21.46,22.4 0 top
C22  22.35,14.15 90 top
C23  14.22,15.8 0 top
C24  22.35,18.21 270 top
C25  17.02,11.86 270 top
C26  14.48,22.4 180 top
C27  23.11,22.4 0 top
D1  29.97,8.56 90 top
D2  29.08,8.56 90 top
D3  13.84,18.97 270 top
D4  8,51.49 270 top
D5  9.53,51.49 270 top
F1  26.86,9.45 90 top
FR1  not placed on the board
FR2  not placed on the board
FR3  not placed on the board
FR4  not placed on the board
J1  29.84,4.75 0 top
J2  18.41,3.86 0 top
J3  38.1,27.74 270 top
J4  10.16,41.71 90 top
J5  10.16,13.77 90 top
J6  38.1,41.71 270 top
J7  10.16,27.74 90 top
J8  38.1,13.77 270 top
K1  8.89,3.23 0 top
K2  38.73,3.23 180 top
L1  22.36,42.21 0 top
L2  22.35,39.17 0 top
L3  22.35,16.18 0 top
L4  18.54,25.07 180 top
P1  not placed on the board
P2  not placed on the board
P3  not placed on the board
P4  not placed on the board
P5  not placed on the board
P6  not placed on the board
P7  not placed on the board
P8  not placed on the board
Q1  18.54,29.12 270 top
Q2  14.99,29.13 270 top
Q4  32.26,22.59 270 top
Q5  27.69,22.59 270 top
R1  27.88,40.5 0 top
R2  30.16,38.53 0 top
R3  15.75,39.17 180 top
R4  13.97,32.05 0 top
R5  16.26,34.72 270 top
R6  16.26,32.5 90 top
R7  22.54,28.5 180 top
R8  26.86,13.64 270 top
R9  31.11,18.97 0 top
R10  32.13,18.97 0 top
R11  29.08,18.97 0 top
R12  33.15,18.97 0 top
R13  30.1,18.97 0 top
R14  34.16,18.97 0 top
R15  17.91,18.97 180 top
R16  15.88,18.97 0 top
R17  14.86,18.97 0 top
R18  16.89,18.97 180 top
R19  14.22,11.86 270 top
R20  14.22,13.13 270 top
R21  16.26,31.42 90 top
R22  13.98,34.21 0 top
R23  16.26,33.58 90 top
R24  14.1,24.94 0 top
R25  30.16,40.5 180 top
R26  28.99,40.49 0 top
R27  16.83,39.17 0 top
R28  15.62,24.43 270 top
R29  15.62,25.58 90 top
U1  21.53,34.47 270 top
U2  28.96,30.15 270 top
U3  31.5,14.02 270 top
U5  17.78,15.04 180 top
U6  18.67,22.15 270 top
X1  29.15,35.36 90 top

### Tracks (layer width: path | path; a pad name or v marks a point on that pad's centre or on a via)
3V3  (via drill 0.3 pad 0.64)
  Top 0.152: R27.1 16.83,40.5 16.13,41.2 14.1,41.2 12.45,42.85 12.45,45.01 10.92,46.53 10.92,52.12 10.16,52.88 8.64,52.88 D4.+
  Top 0.254: U1.4 21.78,37.5 | 21.78,37.58 21.78,37.64 22.1,37.64 22.28,37.46 U1.3 | 21.78,37.5 21.89,37.62 | U1.30 24.45,35.22 | 24.45,35.22 25.13,35.22 25.78,35.86 25.78,36.37 | U1.1 23.28,37.3 23.5,37.52 23.88,37.52 | U1.17 19.78,31.38 | 24.64,35.03 24.64,34.85 24.51,34.72 U1.29 | 24.64,35.04 24.64,35.1 | R1.1 27.69,40.94 26.8,40.06 C3.2 | 21.78,37.58 C9.2 | 21.78,37.58 21.78,37.5 | 24.64,35.03 24.45,35.22 | 24.64,35.03 24.64,35.04 | 24.64,35.04 24.77,35.17 | U1.11 18.11,35.22 v17.4,35.93
  Top 0.508: C10.2 21.39,29.46 v21.34,29.51 19.78,31.07 19.78,31.38
  Top 0.61: 23.88,37.52 24.13,37.52 25.27,38.66 25.27,39.24 26.09,40.06 C3.2 v26.67,39.55 C5.2 C4.2 26.67,37.64 25.78,36.75 25.78,36.37 | C9.2 19.43,38.72 C8.2 v17.88,38.91 17.88,39.06 17.34,39.61 R27.1 | C12.1 v31.88,33.32 | U2.8 32,32.05 32.26,32.31 32.26,32.94 v31.88,33.32 | v31.88,33.32 32.77,33.32 | 32.77,33.32 32.38,32.94 | L4.2 17.64,24.68 16.13,23.16 C19.2 C26.2 14.48,23.29 14.1,23.67 R24.2 | v17.4,35.93 16.76,35.93 C11.2 | 32.77,33.32 32.89,33.32 33.66,34.09 33.66,40.18 v33.53,40.31 | R28.2 14.16,24.43 R24.2 | R24.2 13.53,24.5 12.95,25.07 12.95,26.97 13.97,27.99 Q2.2 13.72,28.24 12.7,29.26 12.7,31.67 13.53,32.5 R4.1 14.92,32.5 v14.99,32.56 15.05,32.5 R6.1
  Bottom 0.61: v26.67,39.55 28.07,40.94 32.89,40.94 v33.53,40.31 | v17.88,38.91 17.4,38.43 v17.4,35.93 17.4,34.47 | v31.88,33.32 31.5,32.94 23.75,32.94 21.72,30.91 | 21.34,30.53 20.95,30.91 | 20.95,30.91 18.16,33.71 | 18.16,33.71 17.4,33.71 | 17.4,33.71 16.89,33.71 | 17.4,34.21 17.4,33.71 | 17.4,34.47 17.4,34.21 | 17.4,34.21 16.89,33.71 | 17.4,34.47 18.16,33.71 | 21.34,30.53 v21.34,29.51 | 21.72,30.91 21.34,30.53 | 20.95,30.91 21.72,30.91 | 16.89,33.71 16.13,33.71 v14.99,32.56
3V3B  (via drill 0.3 pad 0.64)
  Top 0.152: D5.+ 9.65,52.25 10.41,51.49 10.41,47.55 8.26,45.39 v8.26,42.6
  Top 0.61: J5.3 12.05,14.77 v12.06,14.78 | v5.08,28.75 5.1,28.74 J7.3 10.28,28.75 11.75,28.75 v11.87,28.63 | v8.26,42.6 10.15,42.6 J4.3 | J8.3 40.24,12.77 v40.26,12.75 | v40.26,26.72 40.24,26.74 J3.3 37.98,26.72 36.45,26.72 v36.32,26.59 | v40.26,40.69 38.02,40.69 J6.3 | C18.1 v21.08,26.21 20.32,26.97 16.76,26.97 16,27.74 Q2.3
  Bottom 0.61: v12.06,14.78 12.06,26.59 | 12.06,26.59 12.06,27.1 | 12.06,27.1 12.06,27.61 | v5.08,28.75 5.08,39.42 v8.26,42.6 | v40.26,12.75 v40.26,26.72 v40.26,40.69 | 12.57,27.1 20.19,27.1 v21.08,26.21 21.72,25.58 35.31,25.58 v36.32,26.59 | 12.57,27.1 12.06,27.1 | 12.06,27.61 12.57,27.1 | 12.57,27.1 12.06,26.59 | 12.06,27.61 12.06,28.44 v11.87,28.63
ADC  (via drill 0.3 pad 0.64)
  Top 0.152: U1.6 20.78,37.67 v20.65,37.79 | R26.2 29.58,40.04 v29.59,40.06 R25.1
  Bottom 0.152: v29.59,40.06 28.57,40.06 27.3,38.79 25.65,38.79 23.75,36.88 23.75,34.34 22.73,33.32 19.94,33.32 19.05,34.21 19.05,37.01 19.84,37.79 v20.65,37.79
DSW/GPIO16
  Top 0.152: U1.8 19.78,37.17 19.56,37.39 17.08,37.39 R3.1
GND  (via drill 0.3 pad 0.64)
  Top 0.254: 15.74,15.29 15.62,15.29 | 15.62,15.29 15.37,15.04 | 15.37,15.04 15.24,14.91 | 15.24,14.91 C23.2 14.6,15.29 15.62,15.29 | 15.37,15.04 14.61,15.04 | U5.10 15.74,15.29 | 15.74,15.29 15.37,14.91 | 15.37,14.91 15.24,14.91 | 15.37,14.91 14.99,14.53 14.73,14.53 | 14.73,14.53 14.22,14.53 | 14.73,14.53 14.99,14.78 | U5.6 18.03,15.73 v18.24,15.52 | U3.3 32,15.56 v31.47,15.04 | U5.8 17.03,15.91 17.3,15.65 v17.3,15.52 | U6.3 v18.42,22.15 v18.41,22.15 v18.42,22.14 U6.6 | C1.1 26.99,37.07 27.56,37.64 C4.1 | 10.26,45.29 10.26,45.54 v10.16,45.64 | U6.1 19.42,22.26 19.3,22.15 | C2.2 26.23,33.9 26.16,33.96 | ANT1.1 24.9,46.79 24.79,46.68
  Top 0.305: J4.4 10.26,45.29 | U5.8 17.03,17.31 16.89,17.45
  Top 0.61: C15.1 v25.65,16.69 | 21.87,44.27 21.87,46.98 22.04,46.98 22.04,47.1 24.7,47.1 24.7,47.55 ANT1.1 25.08,47.55 25.08,46.47 24.16,45.54
  Bottom 0.203: v28.55,11.23 28.57,11.23 28.83,11.48 28.83,19.46 v28.04,20.24 | 30.23,19.23 30.23,15.14 v30.33,15.04
  other vias: 13.46,21.64 15.24,21.64 16.76,21.89 17.4,22.15 19.68,22.28 20.45,23.04 21.84,23.93 24,24.18 22.99,23.93 24.13,23.16 16.89,19.99 18.8,19.48 21.72,19.48 20.85,19.48 19.99,18.57 24.77,14.4 24.77,13 25.65,15.67 24.77,15.67 26.19,33.99 28.98,33.73 31.9,35.64 31.01,36.65 31.01,37.92 29.62,38.05 26.7,41.86 21.62,40.08 20.6,40.46 18.19,40.46 14.63,36.14 21.51,34.47 20.12,34.47 22.91,34.47 22.91,35.61 21.51,35.61 20.12,35.61 9.6,31.9 10.13,17.7 13.06,13.13 13.06,14.78 13.06,11.86 15.85,11.86 17.75,15.04 31.47,14.02 32.61,14.02 30.33,14.02 32.61,15.04 32.61,13 31.47,13 30.33,13 19.68,11.23 18.8,11.23 27.3,28.24 28.55,6.65 28.55,9.7 30.45,9.7 30.48,6.63 13.34,1.68 14.99,1.68 20.32,1.68 21.84,1.68 28.83,1.55 30.86,1.55 32,1.55 27.69,1.55 16.64,1.68 23.5,1.68 6.1,1.68 11.68,1.68 35.81,4.09 41.66,4.09 4.7,8.28 4.67,14.02 16.64,4.22 21.72,4.22 33.43,8.92 29.11,41.86 38.05,37.8 36.02,8.84 38.18,9.86 21.72,9.3 21.72,6.76 27.13,20.12 4.67,19.1 4.67,24.18 4.17,30.02 4.17,34.34 4.67,40.44 4.67,44.5 42.77,44.5 42.77,39.42 42.77,34.34 42.77,29.26 42.77,24.18 42.77,19.1 42.77,14.02 42.77,8.94 16.48,11.1 13.69,11.1 10.77,36.63 21.62,41.35 23.77,40.08 23.52,38.56 21.87,38.43 12.73,33.86 28.83,27.86 8.2,29.87 7.32,23.27 7.32,18.31 7.32,13.36 37.44,23.42 35.98,24.94 33.25,23.93 30.45,24.56 20.55,27.99 15.15,26.21 12.74,35.99 31.22,40.06 34.9,39.8 32.61,37.52 37.57,19.23 40.11,10.72 15.01,34.75 13.36,40.08 24.85,43.13 26,44.4 20.73,42.11 19.52,47.07 21.42,47.07 24.98,47.07 17.61,47.07 15.84,47.07 13.93,47.07 17.61,45.8 19.52,45.8 24.98,45.8 15.84,45.8 13.93,45.8 19.52,44.4 21.42,44.4 23.96,44.4 17.61,44.4 15.84,44.4 13.93,44.4 20.28,43.13 22.76,43.13 13.93,43.13 32.73,47.07 34.63,47.07 36.66,47.07 30.82,47.07 28.92,47.07 27.01,47.07 30.82,45.8 34.63,45.8 28.92,45.8 26.76,45.8 30.82,44.4 34.63,44.4 28.92,44.4 19.27,41.61 33.36,43.13 27.01,43.13 17.81,42.11 15.27,42.11 31.78,41.86 24.92,41.86 24.92,40.08 23.77,41.86 23.33,47.07 21.42,45.8 23.33,45.8 32.73,45.8 32.73,44.4 18.52,27.99 21.44,27.1 20.55,23.8 36.55,31.93 33.38,32.31 35.53,34.09 34.9,36.63 39.22,35.1 35.92,38.79 6.2,31.8 6.58,34.34 6.45,37.9 8.36,41.33 12.17,41.58 13.06,20.24 13.18,23.55 25.88,19.61 25.12,21.77 26.52,24.69 33.38,21.39 35.03,19.61 37.44,21.89 34.9,21.51 29.57,26.47 31.34,26.47
  pour Bottom (isolate 0.254, rank 6): -0.64,47.29 48.9,47.29 48.9,-0.84 -0.64,-0.84
  pour Top (isolate 0.254, rank 6): -0.64,47.29 48.9,47.29 48.9,-0.84 -0.64,-0.84
  pour Top (isolate 0.254, no thermals): 32.26,33.07 26.29,33.07 25.91,33.45 25.91,39.42 26.16,39.67 32.26,39.67 32.64,39.29 32.64,33.45
  pour Top (isolate 0.254, no thermals): 12.7,3.23 34.29,3.23 34.29,0.43 12.7,0.43
  pour Top (isolate 0.254): 0.38,47.8 5.33,47.8 5.33,43.74 0.38,43.74
  pour Top (isolate 0.254): 42.8,47.93 47.75,47.93 47.75,43.87 42.8,43.87
GPIO4  (via drill 0.3 pad 0.64)
  Top 0.152: U1.16 18.82,32.72 18.54,32.44 18.54,32.05 v18.8,31.8 | J8.2 36.47,14.77 35.94,15.29 35.94,22.91 34.42,24.43 v34.42,27.1
  Bottom 0.152: v18.8,31.8 18.8,31.17 22.86,27.1 v34.42,27.1
GPIO5  (via drill 0.3 pad 0.64)
  Top 0.152: J8.1 36.5,16.77 36.32,16.94 36.32,23.04 35.31,24.05 v35.31,27.74 | U1.24 24.22,32.02 v24.26,32.05
  Bottom 0.152: v24.26,32.05 24.38,32.18 26.04,32.18 29.08,29.13 33.4,29.13 34.8,27.74 v35.31,27.74
HSPICLK/GPIO14
  Top 0.152: J4.1 14.56,38.71 15.37,37.9 16.13,37.9 17.02,37.01 17.78,37.01 18.57,36.22 U1.9
HSPICS/GPIO15
  Top 0.152: R23.2 R5.1 17.53,34.72 18.03,34.22 U1.13
HSPID/GPIO13  (via drill 0.3 pad 0.64)
  Top 0.152: J5.1 8.3,10.77 v8.26,10.72 | J7.2 6.62,26.74 v6.48,26.59 | U1.12 18.04,34.72 17.4,35.36 v11.43,35.36
  Bottom 0.152: v8.26,10.72 6.48,12.5 v6.48,26.59 6.48,30.4 v11.43,35.36
HSPIQ/GPIO12  (via drill 0.3 pad 0.64)
  Top 0.152: J7.1 5.89,24.74 v5.84,24.69 | J4.2 8.79,40.71 8.26,40.17 v8.26,37.9 8.76,37.39 16.13,37.39 16.89,36.63 17.53,36.63 18.43,35.72 U1.10
  Bottom 0.152: v5.84,24.69 5.84,30.28 8.26,32.69 v8.26,37.9
N$1  (via drill 0.3 pad 0.64)
  Top 0.152: R2.1 30.8,38.98 v30.99,38.79 | U1.31 24.59,35.72 v24.79,35.92
  Bottom 0.152: v30.99,38.79 29.21,38.79 26.34,35.92 v24.79,35.92
N$2
  Top 0.254: X1.3 27.3,35.8 C1.2 26.48,35.8 25.91,35.23 25.84,35.17 24.9,34.22 U1.28
N$3
  Top 0.254: X1.1 30.16,34.28 29.34,35.1 27.3,35.1 C2.1 26.1,34.78 25.03,33.72 U1.27
N$4
  Top 0.152: U1.7 20.28,37.35 19.85,37.77 17.27,37.77 16.83,38.21 R27.2
N$5
  Top 0.254: U1.2 22.78,39.15 L2.2 C7.1
N$6
  Top 0.254: C7.2 22.8,42.2 L1.2 22.86,42.21 24.74,44.09 arc45 26.08,47.33 ANT1.2
N$7  (via drill 0.3 pad 0.64)
  Top 0.152: R24.1 14.1,26.72 15.11,27.74 v15.11,28.24 14.99,28.37 14.99,29.13 14.1,30.02 Q2.1 | Q1.3 18.68,29.12 v18.67,29.13
  Bottom 0.152: v15.11,28.24 17.78,28.24 v18.67,29.13
N$8
  Top 0.152: U3.26 34.51,14.52 34.8,14.81 34.8,16.31 33.53,17.58 32.51,17.58 32.13,17.96 R10.2
N$9
  Top 0.152: J6.1 36.45,44.71 32.69,40.94 R25.2
N$10
  Top 0.152: R7.1 24.83,28.05 25.27,27.61 27.56,27.61 29.15,29.2 29.21,29.26 29.46,29.51 U2.6
N$11  (via drill 0.3 pad 0.64)
  Top 0.152: R23.1 15.37,33.13 13.14,33.13 12.06,32.05 12.06,30.11 v11.68,29.73 | Q1.1 18.27,30.01 v18.41,30.15
  Bottom 0.152: v18.41,30.15 18.16,29.9 11.85,29.9 v11.68,29.73
N$12
  pour Top (isolate 0.254, no thermals): 28.45,3.73 28.7,3.73 28.8,3.84 28.8,4.91 arc45 28.45,5.77 27.81,6.4 27.81,8.69 27.69,8.81 25.91,8.81 25.78,8.69 25.78,6.27 26.67,5.38 arc45 27.28,5.13 28.04,5.13 28.32,4.85 28.32,3.86
N$13
  Top 0.152: U3.5 31,17.19 30.2,17.98 29.63,17.98 R11.2
N$14  (via drill 0.3 pad 0.64)
  Top 0.152: R21.1 v15.11,31.42 | v11.68,32.56 11.68,32.69 7.24,37.13 7.24,45.52 8,46.28 D4.-
  Bottom 0.152: v15.11,31.42 14.86,31.42 13.72,32.56 v11.68,32.56
N$15  (via drill 0.3 pad 0.64)
  Top 0.152: D2.1 v29.08,7.42 29.34,7.16 29.34,5.26 29.2,5.12 J1.2 | v29.08,20.24 R11.1
  Bottom 0.152: v29.08,7.42 29.34,7.67 29.34,19.99 v29.08,20.24
N$16  (via drill 0.3 pad 0.64)
  Top 0.152: D1.1 v29.97,7.42 29.65,7.1 29.65,5.26 29.84,5.07 J1.3 | R13.1 v30.1,20.24
  Bottom 0.152: v29.97,7.42 29.97,7.48 29.72,7.73 29.72,19.86 v30.1,20.24
N$17
  Top 0.152: U3.4 31.5,17.13 R13.2
N$18  (via drill 0.3 pad 0.64)
  Top 0.152: R14.1 v34.16,20.24 | Q5.1 27.62,23.48 v27.69,23.55
  Bottom 0.152: v34.16,20.24 33.27,20.24 29.97,23.55 v27.69,23.55
N$19
  Top 0.152: U3.9 27.67,15.02 C13.2 R8.1
N$20
  Top 0.152: U3.25 34.67,14.02 35.18,14.53 35.18,16.5 R12.2
N$22
  Top 0.152: R22.1 10.22,34.66 7.62,37.26 7.62,45.26 9.53,47.17 D5.-
N$23  (via drill 0.3 pad 0.64)
  Top 0.152: U3.24 34.68,13.52 35.56,14.4 35.56,17.07 v34.67,17.96 34.16,18.47 R14.2 | Q4.2 v31.24,20.88
  Bottom 0.152: v31.24,20.88 31.75,20.88 v34.67,17.96
N$24  (via drill 0.3 pad 0.64)
  Top 0.152: U3.28 34.27,15.52 34.42,15.67 34.42,16.05 33.27,17.2 32.26,17.2 v31.5,17.96 31.24,17.96 31.11,18.08 R9.2 | Q5.2 27.47,21.7 v27.56,21.79
  Bottom 0.152: v31.5,17.96 31.5,19.74 29.44,21.79 v27.56,21.79
N$25
  Top 0.152: R9.1 31.11,20.12 30.23,21.01 30.23,23.16 30.54,23.48 Q4.1
N$26
  Top 0.254: U5.3 20.57,15.29 L3.1
  pour Top (isolate 0.254, no thermals): 18.8,16.81 18.8,15.42 18.92,15.29 21.84,15.29 21.97,15.42 21.97,16.81 21.84,16.94 18.92,16.94
N$28
  Top 0.254: U5.16 18.53,12.84 | 18.53,12.84 18.53,12.74 18.41,12.62 | 18.41,12.62 18.29,12.5 | U5.14 17.53,11.93 C25.1 | 18.29,12.5 17.78,12.5 | 18.41,12.62 17.78,12.62 | 18.53,12.84 18.29,12.6 | 18.29,12.5 17.91,12.12
  pour Top (isolate 0.254, no thermals): 17.27,7.04 17.98,7.04 18.16,7.22 18.16,12.62 18.03,12.75 17.4,12.75 17.14,12.5 17.14,7.16
N$29
  Top 0.305: U6.2 18.92,23.8
  pour Top (isolate 0.254, no thermals): 19,22.66 18.8,22.66 18.75,22.71
  pour Top (isolate 0.254, no thermals): 18.8,23.55 19.37,23.55 19.88,24.05 19.88,25.83 19.81,25.9 19.05,25.9 18.99,25.83 18.99,24.12 18.73,23.86 18.73,23.61
N$30
  Top 0.152: R17.1 14.8,19.42 14.61,19.23 14.54,19.16 13.88,18.51 D3.-
N$31
  Top 0.152: U5.9 15.76,15.79 15.37,16.18 15.37,18.02 R17.2
N$32  (via drill 0.3 pad 0.64)
  Top 0.305: U6.4 17.92,23.68 v18.03,23.8 | v16.64,24.82 16.26,24.43 R28.1 R29.2
  Bottom 0.305: v18.03,23.8 17.02,24.82 v16.64,24.82
N$33
  Top 0.152: U5.7 17.53,17.89 R18.1 R16.2
N$34
  Top 0.152: U5.11 15.8,14.79 14.99,13.97 14.99,13.51 14.67,13.2 R20.1
N$36
  Top 0.152: U5.12 15.76,14.29 15.37,13.89 15.37,12.56 R19.1
N$37
  Top 0.254: U5.5 18.53,17.91 R15.1
RST  (via drill 0.3 pad 0.64)
  Top 0.152: C6.2 28.63,38.99 | 28.63,38.99 28.52,38.99 v28.45,38.91 28.45,39.17 | 27.81,40.06 R1.2 28.45,39.48 28.45,39.17 | 28.63,38.99 28.45,39.17 | K2.4 39.29,2.29 v39.24,2.34 39.19,2.29 K2.3 | U1.32 24.23,36.22 25.86,37.85 v25.86,38.13 | R3.2 v15.75,40.31 | Q4.3 34.23,22.59 v34.29,22.66
  Bottom 0.152: v39.24,2.34 39.24,22.4 | 39.24,22.4 39.24,22.66 | 39.24,22.66 39.24,22.91 | 39.24,22.91 39.24,33.96 33.78,39.42 28.96,39.42 v28.45,38.91 27.66,38.13 v25.86,38.13 25.86,38.1 24.13,36.37 24.13,34.21 22.86,32.94 19.81,32.94 18.54,34.21 18.54,39.04 17.27,40.31 v15.75,40.31 | v34.29,22.66 38.86,22.66 38.99,22.66 | 38.99,22.66 39.24,22.66 | 38.99,22.66 39.24,22.91 | 38.99,22.66 39.24,22.4
SPICLK/SD_CLK  (via drill 0.3 pad 0.64)
  Top 0.152: U1.21 21.78,31.49 22.48,30.78 24.26,30.78 v24.51,30.53 | R7.2 23.18,28.94 v23.24,29.01
  Bottom 0.152: v23.24,29.01 23.24,29.26 v24.51,30.53
SPICS0/SD_CMD
  Top 0.152: U1.20 21.28,31.48 22.35,30.4 23.75,30.4 24.26,29.9 25.27,29.9 25.53,30.15 27.05,30.15 27.3,30.4 27.3,31.8 27.05,32.05 U2.1
SPICS2/GPIO0  (via drill 0.3 pad 0.64)
  Top 0.152: U1.15 18.69,33.22 18.03,32.56 v18.03,31.42 | K1.3 8.97,4.17 v8.89,4.24 8.81,4.17 K1.4 | Q5.3 v28.7,26.47 | R4.2 13.97,31.23 v13.78,31.04
  Bottom 0.152: v8.89,4.24 8.89,28.63 11.3,31.04 v13.78,31.04 14.54,30.28 16.26,30.28 17.4,31.42 v18.03,31.42 22.99,26.47 v28.7,26.47
SPID/SD_D1  (via drill 0.3 pad 0.64)
  Top 0.152: U1.23 22.78,31.63 22.99,31.42 25.02,31.42 v25.15,31.55 | U2.5 v30.48,28.24
  Bottom 0.152: v25.15,31.55 26.04,31.55 29.34,28.24 v30.48,28.24
SPIHD/HSPIHD/SD_D2
  Top 0.152: U1.18 20.28,31.46 22.1,29.64 23.5,29.64 24.13,29.01 28.32,29.01 29.4,30.09 29.46,30.15 30.1,30.78 U2.7
SPIQ/SD_D0
  Top 0.152: U1.22 22.28,31.55 22.73,31.09 24.84,31.09 25.15,30.78 U2.2
SPIWP/HSPIWP/SD_D3
  Top 0.152: U1.19 20.78,31.47 22.23,30.02 23.62,30.02 24.13,29.51 U2.3
U0RXD/SPICS1/GPIO3  (via drill 0.3 pad 0.64)
  Top 0.152: R10.1 32.13,26.34 35.43,29.64 35.43,30.53 | J3.1 35.64,30.74 | 35.61,30.74 35.48,30.74 35.43,30.78 | 35.43,30.78 v35.43,30.91 35.61,30.74 | 35.43,30.78 35.43,30.53 | 35.64,30.74 35.61,30.74 | 35.64,30.74 35.43,30.53 | U1.25 25.88,32.72 26.04,32.56 27.18,32.56 28.07,31.67 v28.07,31.42
  Bottom 0.152: v28.07,31.42 28.57,30.91 v35.43,30.91
U0TXD/GPIO1  (via drill 0.3 pad 0.64)
  Top 0.152: R12.1 33.15,19.99 32.44,20.7 32.44,26.14 34.67,28.37 v36.2,28.37 37.63,28.37 J3.2 | U1.26 25.89,33.22 26.16,32.94 28.25,32.94 v29.59,31.6
  Bottom 0.152: v29.59,31.6 35.76,31.6 36.2,31.17 v36.2,28.37
U1TXD/GPIO2  (via drill 0.3 pad 0.64)
  Top 0.152: U1.14 18.43,33.72 17.35,32.64 v17.35,32.44 17.29,32.5 16.76,32.5 | J5.2 8.27,12.77 v8.26,12.75 | R6.2 16.76,32.5 | R21.2 16.7,32.44 16.76,32.5
  Bottom 0.152: v8.26,12.75 8.26,28.63 11.56,31.93 13.72,31.93 14.99,30.66 16,30.66 17.35,32 v17.35,32.44
VDD  (via drill 0.3 pad 0.64)
  Top 0.254: U3.6 30.5,16.93 | 30.5,16.93 30.5,17.18 30.23,17.45 | 30.23,17.45 29.97,17.45 | 30.23,17.45 30.1,17.58 | 30.5,16.93 30.43,16.93 30.04,17.32
  Top 0.406: R8.2 v26.42,13 | C16.2 27.05,18.34 v26.54,17.83
  Top 0.61: 29.97,17.45 28.45,17.45 28.07,17.83 C17.2 C16.2
  Bottom 0.406: v26.54,17.83 26.54,13.13 v26.42,13
VSYS  (via drill 0.3 pad 0.64)
  Top 0.254: U5.15 18.03,13.89 18.43,14.29 U5.1 19.62,14.29 19.74,14.17 | D3.+ 13.84,19.86 14.61,20.62 17.4,20.62 17.66,20.62 | 17.66,20.62 17.92,20.88 | 17.66,20.62 17.91,20.62
  Top 0.305: U6.5 17.92,20.88 17.92,20.74 | 19.68,20.62 19.56,20.5 18.16,20.5 17.92,20.74 | 19.36,20.6 19.13,20.37 18.11,20.37 17.92,20.56 17.92,20.74
  other vias: 19.15,12.9 19.63,12.5 23.11,19.48 23.75,19.48
  pour Top (isolate 0.254, no thermals): 19.94,12.24 19.94,14.15 19.81,14.27 18.92,14.27 18.8,14.15 18.8,12.24 18.92,12.12 19.81,12.12
  pour Top (isolate 0.254, no thermals): 24,15.42 22.86,15.42 22.73,15.54 22.73,20.12 22.61,20.24 18.92,20.24 18.8,20.37 18.8,21.55 18.93,21.69 20.7,21.69 20.95,22.02 23.75,22.02 24.13,21.64 24.13,15.54
  pour Bottom (isolate 0.254, no thermals): 18.92,13.26 19.43,13.26 19.94,12.75 22.23,12.75 22.73,13.26 22.73,19.61 22.99,19.86 24,19.86 24.13,19.74 24.13,12.62 22.99,11.48 19.05,11.48 18.8,11.73 18.8,13.13
VUSB  (via drill 0.3 pad 0.64)
  Top 0.254: U5.2 20.82,14.79 C22.1
  Top 0.61: R16.1 v15.88,19.99
  Bottom 0.61: v15.88,19.99 15.88,17.96 | 15.88,17.96 15.88,17.32 | 15.88,17.96 15.37,17.45 | 15.88,17.96 16.38,17.45
  other vias: 26.8,11.68 27.43,11.68 27.97,15.65 27.97,16.33 20.62,14.53 20.62,13.89 13.82,17.53 14.45,17.53
  pour Top (isolate 0.254, no thermals): 27.56,10.08 20.57,10.08 20.32,10.34 20.32,14.2 19.86,14.66 19.05,14.66 18.98,14.73 18.98,14.84 19.05,14.91 21.79,14.91 21.97,14.73 21.97,12.15 22.25,11.86 27.63,11.86 27.81,11.68 27.81,10.34
  pour Top (isolate 0.254, no thermals): 29.72,15.93 30.1,15.93 30.23,16.05 30.23,16.81 30.1,16.94 27.05,16.94 26.92,16.81 26.92,15.42 27.05,15.29 29.46,15.29 29.59,15.42 29.59,15.8
  pour Bottom (isolate 0.254, no thermals): 28.45,12.24 27.43,11.23 26.54,11.23 26.29,11.48 26.29,12.32 27.18,13.21 27.18,16.64 27.36,16.81 28.27,16.81 28.45,16.64
  pour Bottom (isolate 0.254, no thermals): 21.84,16.3 21.84,13.64 21.72,13.51 20.32,13.51 20.19,13.64 20.19,15.67 19.68,16.18 13.46,16.18 13.34,16.31 13.34,17.7 13.46,17.83 20.31,17.83
  pour Top (isolate 0.254, no thermals): 14.86,16.18 13.34,16.18 13.21,16.31 13.21,17.7 13.34,17.83 14.73,17.83 14.99,17.58 14.99,16.31
(copper drawn outside any net)
  shapes: Bottom circle x1

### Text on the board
Bottom: FCC ID: Z4T-WIOLINK | A | Model: Wio Link | IC: 21046-WIOLINK
tPlace: + | - | BAT
tNames: BLUE | RED | GND | A0 | 3V3 | NC | 12 | Digital0 | 3V3 | Analog | 14 | GND | GND | RX | 3 | 1 | 3V3 | TX | 13 | 3V3 | UART | Digital1 | 12 | GND | CH | GND | 5 | 3V3 | 4 | I2C | 2 | 3V3 | Digital2 | 13 | GND | CONFIG | RESET

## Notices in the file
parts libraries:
moudle-new: This work is licensed under the Creative Commons Attribution 4.0 International License.
To view a copy of this license,visit:
http://creativecommons.org/licenses/by-sa/4.0
moudle-new: CC-BY-SA
